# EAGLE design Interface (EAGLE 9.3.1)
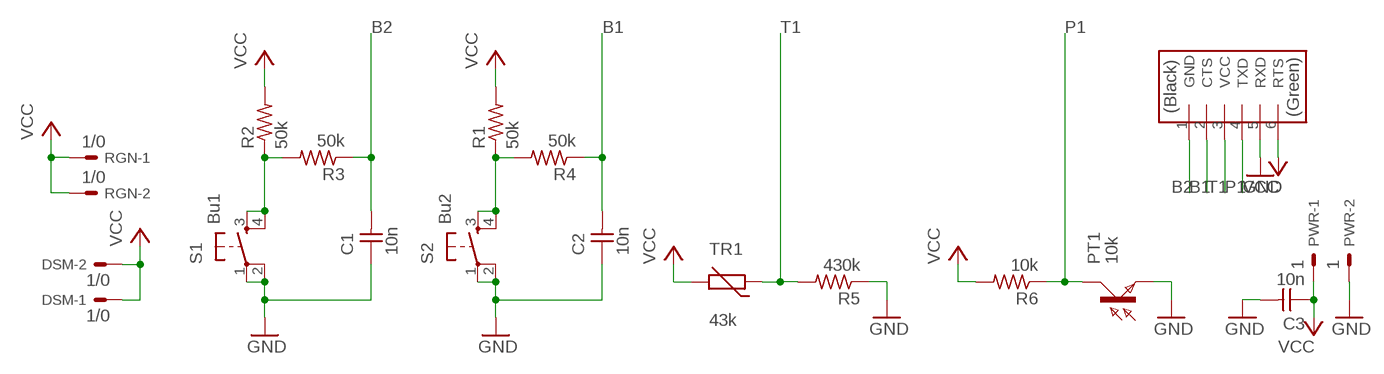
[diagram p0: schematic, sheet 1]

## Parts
C1  10n  CAP-UNPOLARIZEDFAB  [C1206FAB]
C2  10n  CAP-UNPOLARIZEDFAB  [C1206FAB]
C3  10n  CAP-UNPOLARIZEDFAB  [C1206FAB]
DSM  1/0  KK-156-2  [KK-156-2]
PT1  10k  PHOTOTRANSISTOR-NPN1206  [OP1206]
PWR  1  KK-156-2  [KK-156-2]
R1  50k  RES-US1206FAB  [R1206FAB]
R2  50k  RES-US1206FAB  [R1206FAB]
R3  50k  RES-US1206FAB  [R1206FAB]
R4  50k  RES-US1206FAB  [R1206FAB]
R5  430k  RES-US1206FAB  [R1206FAB]
R6  10k  RES-US1206FAB  [R1206FAB]
RGN  1/0  KK-156-2  [KK-156-2]
S1  Bu1  6MM_SWITCH6MM_SWITCH  [6MM_SWITCH]
S2  Bu2  6MM_SWITCH6MM_SWITCH  [6MM_SWITCH]
TR1  43k  THERMISTOR_R-7,5  [R-7,5]
U$1  FTDI-SMD-HEADER  [1X06SMD]

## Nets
B1: C2.2 R4.1 U$1.2(CTS)
B2: C1.2 R3.1 U$1.1(GND)
GND: C1.1 C2.1 C3.2 PT1.EMITTER(E) PWR.2 R5.1 S1.1(P) S1.2(P1) S2.1(P) S2.2(P1) U$1.5(RXD)
N$1: R2.1 R3.2 S1.3(S) S1.4(S1)
N$3: R1.1 R4.2 S2.3(S) S2.4(S1)
P1: PT1.COLLECTOR(C) R6.1 U$1.4(TXD)
T1: R5.2 TR1.1 U$1.3(VCC)
VCC: C3.1 DSM.1 DSM.2 PWR.1 R1.2 R2.2 R6.2 RGN.1 RGN.2 TR1.2 U$1.6(RTS)

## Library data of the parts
C1-C3 = fab:CAP-UNPOLARIZED
DSM PWR RGN = con-molex:KK-156-2: KK 156 HEADER; MF: MOLEX; OC_FARNELL: unknown; OC_NEWARK: unknown
PT1 = fab:PHOTOTRANSISTOR-NPN
R1-R6 = fab:RES-US: Resistor (US Symbol)
S1 S2 = fab:6MM_SWITCH: OMRON SWITCH
TR1 = discrete:THERMISTOR_: Thermo Resistor
U$1 = fab:FTDI-SMD-HEADER

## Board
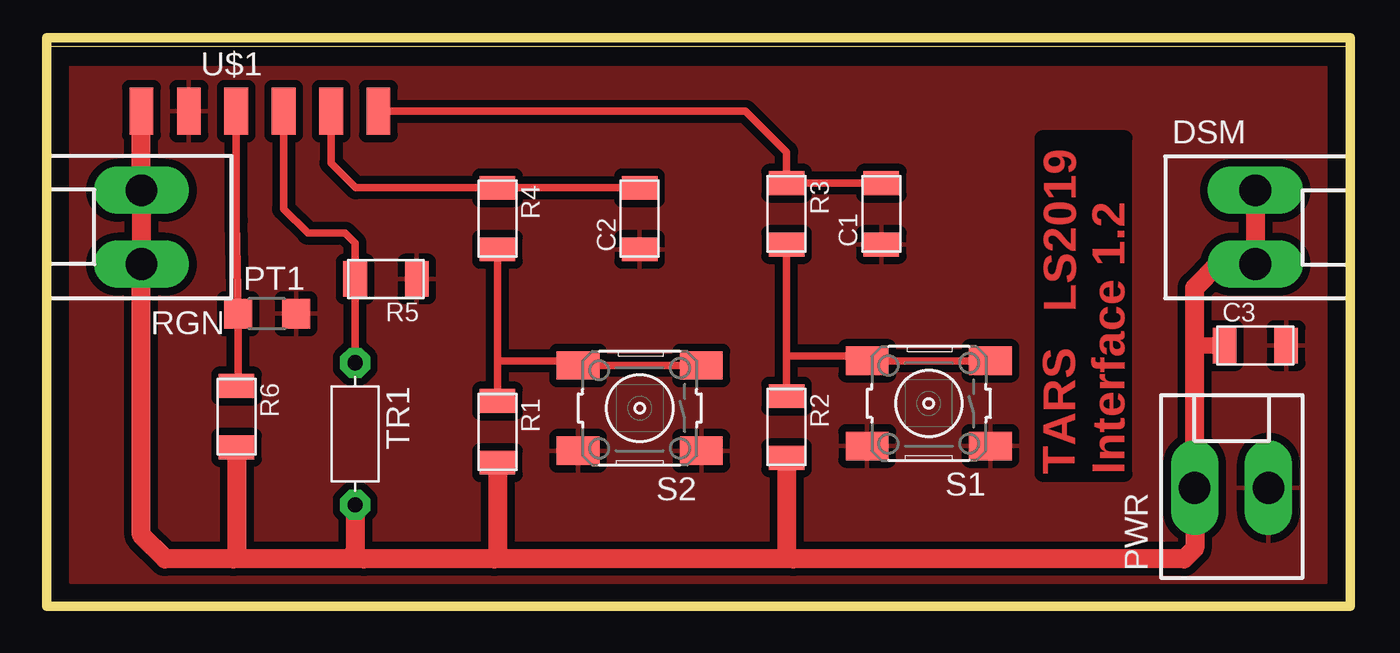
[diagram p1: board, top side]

Size 70 x 30 mm. Coordinates in mm from the lower left corner, seen from the top.
Outline: 0,0 70,0 70,30 0,30 0,0
Copper layers (1*16): Top 0.035mm / dielectric 1.5mm / Bottom 0.035mm
Design rules "default *": minimum track width 16mil, minimum drill 0.35mm, track to track 16mil, track to pad 16mil, pad to pad 16mil, via to via 16mil, smd to smd 16mil, copper to edge 40mil, drill to drill 16mil, minimum pad ring 10mil, minimum via ring 8mil, stop-mask expansion 16mil, vias tented up to drill 0mil, thermal gap 16mil
Milling: 4 lines

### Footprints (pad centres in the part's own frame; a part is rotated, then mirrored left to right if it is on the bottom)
C1206FAB = smd 1.27 x 1.905: 1 -1.651,0; 2 1.651,0
KK-156-2 = drill 1.7 pad 2.184 long: 1 -1.98,0; 2 1.98,0
OP1206 = smd 1.5 x 1.6: COLLECTOR -1.55,0; EMITTER 1.55,0
R1206FAB = smd 1.27 x 1.905: 1 -1.651,0; 2 1.651,0
6MM_SWITCH = smd 2.286 x 1.524: 1 -3.302,2.286; 2 3.302,2.286; 3 -3.302,-2.286; 4 3.302,-2.286
R-7,5 = drill 0.813 pad 1.6 octagon: 1 -3.81,0; 2 3.81,0
1X06SMD = smd 2.54 x 1.27: 1 0,6.35; 2 0,3.81; 3 0,1.27; 4 0,-1.27; 5 0,-3.81; 6 0,-6.35

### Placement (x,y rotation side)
C1  44.73,21.03 90 top
C2  31.78,20.78 90 top
C3  64.77,13.97 0 top
DSM  64.77,20.32 270 top
PT1  11.81,15.68 0 top
PWR  63.5,6.35 0 top
R1  24.16,9.35 270 top
R2  39.65,9.6 270 top
R3  39.65,21.03 270 top
R4  24.16,20.78 270 top
R5  18.18,17.54 180 top
R6  10.18,10.16 270 top
RGN  5.08,20.32 90 top
S1  47.27,10.87 180 top
S2  31.78,10.62 180 top
TR1  16.53,9.24 270 top
U$1  11.43,26.54 270 top

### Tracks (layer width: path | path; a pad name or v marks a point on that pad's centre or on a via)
B1
  Top 0.406: C2.2 R4.1 16.57,22.43 15.24,23.76 U$1.2
B2
  Top 0.406: C1.2 R3.1 39.65,24.35 37.46,26.54 U$1.1
GND
  pour Top: 1.27,29.21 1.27,1.27 68.58,1.27 68.58,29.21
N$1
  Top 0.406: S1.3 S1.4 43.72,13.41 39.65,13.41 | R2.1 39.65,13.41 | 39.65,13.41 R3.2
N$3
  Top 0.406: S2.3 S2.4 28.22,13.16 24.16,13.16 | R1.1 24.16,13.16 | 24.16,13.16 R4.2
P1
  Top 0.406: R6.1 10.26,11.81 PT1.COLLECTOR 10.16,20.68 U$1.4
T1
  Top 0.406: TR1.1 R5.2 16.53,19.47 16,20 14,20 12.7,21.3 U$1.3
VCC
  Top 0.406: 10.18,2.72 10,2.54 | 16.53,3.01 17,2.54 | 24.16,2.7 24,2.54 | R2.2 39.95,7.95 40,8 | 39.65,2.89 40,2.54
  Top 0.889: C3.1 61.52,13.97
  Top 1.016: DSM.1 DSM.2 62.79,18.34 61.52,17.07 61.52,13.97 PWR.1 61.52,3.1 60.96,2.54 40,2.54 24,2.54 17,2.54 10,2.54 6.35,2.54 5.08,3.81 RGN.1 RGN.2 U$1.6 | R6.2 10.18,2.72 | TR1.2 16.53,3.01 | R1.2 24.16,2.7 | R2.2 39.65,2.89

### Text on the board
Top: LS2019 | TARS / Interface 1.2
